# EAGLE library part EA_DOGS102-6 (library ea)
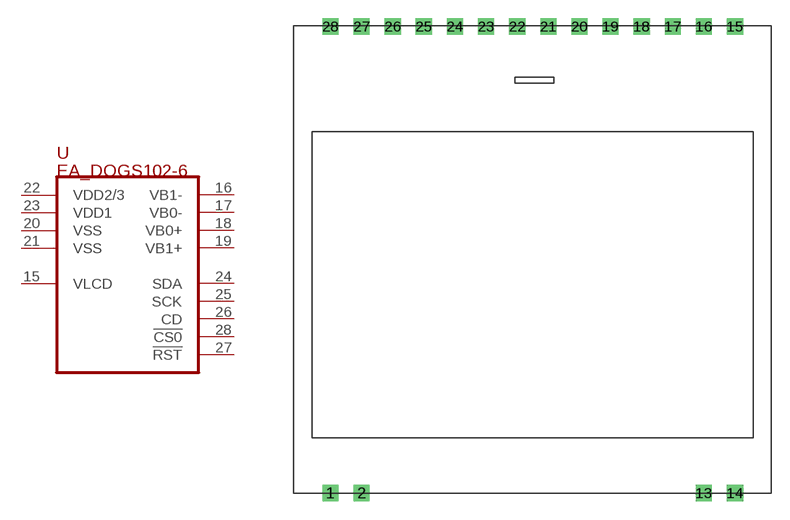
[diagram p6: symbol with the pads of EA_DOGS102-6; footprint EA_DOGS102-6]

Designator prefix -

## EA_DOGS102-6  [EA_DOGS102-6]
15  VLCD
16  VB1-
17  VB0-
18  VB0+
19  VB1+
20  VSS
21  VSS
22  VDD2/3  pwr
23  VDD1  pwr
24  SDA
25  SCK  in
26  CD
27  !RST!  in
28  !CS0!  in

## Footprint EA_DOGS102-6 (pad centres in mm)
EA DOGS102-6 Grafikdisplay COG 102x64 Pixel inkl.Kontroller Hersteller: ELECTRONIC ASSEMBLY GmbH http://www.lcd-module.de
drill 0.813 square: 1 0,0; 2 2.54,0; 13 30.48,0; 14 33.02,0; 15 33.02,38.1; 16 30.48,38.1; 17 27.94,38.1; 18 25.4,38.1; 19 22.86,38.1; 20 20.32,38.1; 21 17.78,38.1; 22 15.24,38.1; 23 12.7,38.1; 24 10.16,38.1; 25 7.62,38.1; 26 5.08,38.1; 27 2.54,38.1; 28 0,38.1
